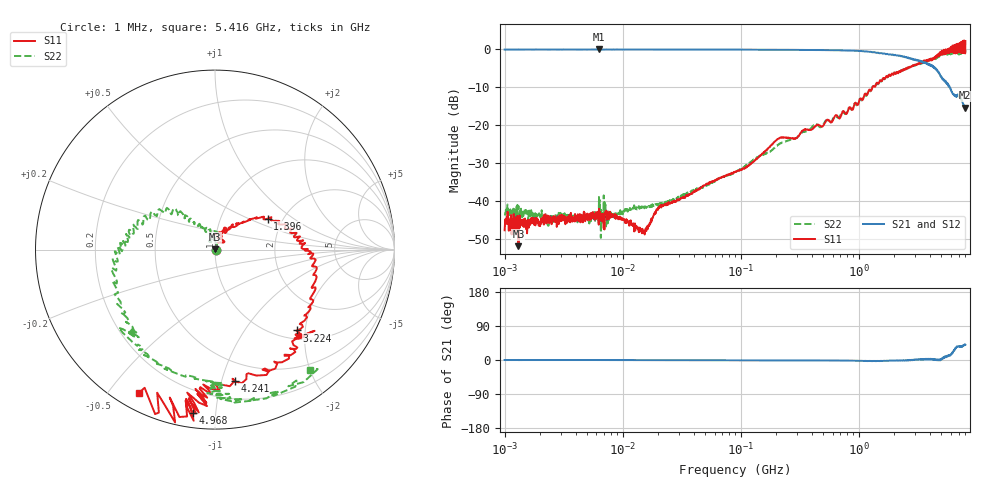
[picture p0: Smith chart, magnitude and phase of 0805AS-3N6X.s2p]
!s-Parameter Generated by FASTRON Sdn. Bhd.
!FASTRON P/N : 0805AS-3N6X
!Keysight Technologies: E5071C_MY46733604_B.14.02
!Date: Mon Jun 15 12:46:45 2026
!Version  :Rev01  Mon Jun 15 12:46:45 2026
!Data & Calibration Information:
!Freq  S11:SOLT2(ON)  S21:SOLT2(ON)  S12:SOLT2(ON)  S22:SOLT2(ON)
!PortZ  Port1:50+j0  Port2:50+j0
!When reading reference impedance value at option line is always used.
! Remarks : This data is being provided solely for informational purposes.
# Hz S dB R 50
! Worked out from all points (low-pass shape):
!   1601 points, 1 MHz to 8 GHz, reference 50 ohm
!   highest |S21| = -0.03 dB at 6.301 MHz (marker M1); lowest = -15.4 dB at 7.923 GHz (marker M2)
!   |S21| within 3 dB of the highest: start of sweep to 3.227 GHz; 3.281 GHz to 3.311 GHz (29.73 MHz wide, 0.902 % of centre)
!   lowest |S11| = -52.0 dB at 1.31 MHz (marker M3), VSWR 1.01, Z = 50.1 + j0.215 ohm
!   |S11| at or under -10 dB: start of sweep to 1.307 GHz
!   |S22| runs from -49.8 to -0.1 dB; largest |S21 - S12| = 0.0073
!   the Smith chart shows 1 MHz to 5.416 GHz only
!   S11 on the Smith chart (normalised r, x): 1 MHz: 1.01, -0.00; 1.396 GHz: 1.67, +0.65; 3.224 GHz: 1.18, -1.80; 4.241 GHz: 0.34, -1.10; 4.968 GHz: 0.07, -0.87; 5.416 GHz: 0.07, -0.60
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1000000  -47.80 -8.8  -0.07 -0.1  -0.05 -0.1  -43.60 1.8
1310238  -52.00 58.4  -0.10 0.2  -0.07 -0.1  -41.40 -17.0
4479405  -44.60 4.3  -0.06 -0.0  -0.06 -0.1  -44.80 8.8
6301378  -42.10 14.8  -0.03 -0.4  -0.00 -0.1  -39.00 26.4
1.492352e7  -48.40 10.1  -0.05 -0.1  -0.07 -0.1  -41.90 21.1
2.00676e7  -41.90 31.9  -0.06 -0.2  -0.07 -0.1  -41.00 41.8
8.994653e7  -32.30 70.2  -0.08 -0.5  -0.09 -0.4  -32.40 69.0
2.111884e8  -23.50 39.4  -0.13 -0.6  -0.14 -0.7  -25.10 124.0
4.006501e8  -21.10 89.4  -0.18 -1.0  -0.19 -1.0  -20.60 80.7
1.395953e9  -9.37 30.5  -0.90 -3.0  -0.91 -3.1  -9.20 139.0
1.7949e9  -6.83 11.9  -1.39 -1.9  -1.39 -2.1  -6.76 159.0
2.486897e9  -5.07 -5.2  -2.11 -0.4  -2.16 -0.7  -5.06 -179.0
3.223742e9  -3.87 -44.7  -3.01 1.0  -3.04 1.0  -3.90 -135.0
3.710194e9  -3.13 -52.5  -3.64 1.0  -3.61 1.1  -3.26 -126.0
4.240668e9  -2.62 -81.5  -4.60 2.5  -4.57 2.3  -2.76 -99.1
4.968456e9  -0.73 -97.8  -7.07 0.4  -7.06 0.3  -1.41 -83.7
5.416325e9  -0.87 -118.0  -8.56 9.4  -8.58 9.1  -1.35 -51.6
6.110812e9  0.27 -130.0  -11.20 17.1  -11.20 16.1  -1.13 -31.1
6.534915e9  1.18 -127.0  -12.20 30.2  -12.20 29.2  -0.47 3.4
6.959019e9  -0.71 -148.0  -12.40 35.9  -12.30 35.1  -0.88 42.1
7.92289e9  1.33 -169.0  -15.40 40.4  -15.20 39.8  -0.13 75.2
8e9  2.20 178.0  -15.40 40.2  -15.20 39.7  -0.24 72.4
